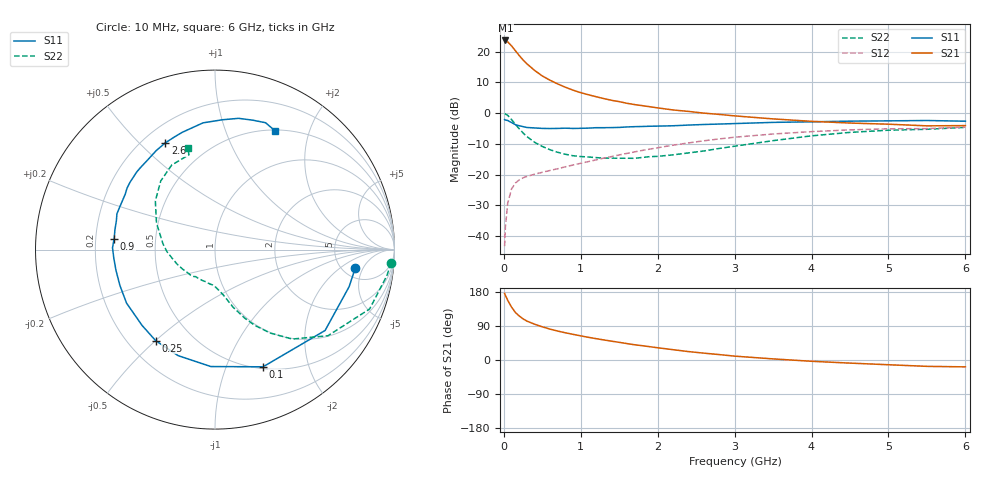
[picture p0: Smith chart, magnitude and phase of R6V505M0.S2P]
! SIEMENS Small Signal Semiconductors
! BFR193
! Si NPN RF Bipolar Junction Transistor in SOT23
! VCE = 0.5 V  IC = 5 mA
! Common Emitter S-Parameters:  May  1996
# GHz  S  MA  R  50
!  f  S11  S21  S12  S22
! GHz  MAG  ANG  MAG  ANG  MAG  ANG  MAG  ANG
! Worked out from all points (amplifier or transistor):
!   36 points, 10 MHz to 6 GHz, reference 50 ohm
!   highest |S21| = 23.6 dB at 20 MHz (marker M1)
!   |S21| within 3 dB of that: start of sweep to 139.3 MHz
!   unconditionally stable (mu >= 1): 849.4 MHz to 2.434 GHz; 5.47 GHz to end of sweep
!   at 250 MHz: K = 0.44, MSG = 19.2 dB, |S12| = -21.0 dB
!   at 1.4 GHz: K = 1.10, MAG = 7.3 dB, |S12| = -14.1 dB
!   at 6 GHz: K = 1.01, MAG = -0.2 dB, |S12| = -4.5 dB
!   S11 on the Smith chart (normalised r, x): 10 MHz: 6.44, -3.54; 100 MHz: 0.52, -1.36; 250 MHz: 0.31, -0.50; 900 MHz: 0.28, +0.05; 2.6 GHz: 0.29, +0.60; 6 GHz: 0.51, +1.50
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0.01  0.7877 -7.6  15.21 175.7  0.0069 85.6  0.9842 -4.3
0.02  0.7755 -15.4  15.22 170.6  0.014 81.1  0.9682 -8.7
0.05  0.7611 -36.3  14.45 157.7  0.0342 71.8  0.9228 -21.0
0.1  0.7058 -67.7  12.43 139.6  0.0585 59.0  0.7916 -37.3
0.15  0.652 -92.0  10.37 125.5  0.0734 50.2  0.6584 -49.2
0.2  0.6254 -109.2  8.661 116.1  0.0824 45.0  0.5575 -56.5
0.25  0.6055 -123.1  7.337 108.5  0.0891 42.2  0.478 -62.2
0.3  0.5861 -133.9  6.351 102.7  0.0938 40.8  0.417 -66.5
0.4  0.576 -148.8  4.962 94.4  0.102 40.1  0.3369 -72.5
0.5  0.5663 -159.3  4.031 87.5  0.1095 40.7  0.288 -76.3
0.6  0.5637 -168.3  3.438 81.5  0.1173 41.9  0.2549 -79.9
0.7  0.5659 -175.4  2.992 76.4  0.1252 43.5  0.2317 -83.9
0.9  0.5652 173.8  2.367 67.7  0.1438 46.1  0.2033 -90.7
1.1  0.5723 163.8  1.994 59.8  0.1636 47.8  0.1941 -97.9
1.3  0.5815 155.6  1.727 52.9  0.1864 48.7  0.186 -106.1
1.6  0.598 145.0  1.449 43.3  0.2222 48.9  0.1855 -120.5
2.2  0.6249 126.8  1.129 27.2  0.3022 44.9  0.2106 -148.9
2.6  0.6557 115.0  1.003 18.1  0.356 40.2  0.2432 -168.5
3.5  0.7093 95.4  0.808 2.9  0.4593 26.2  0.3579 155.6
4.5  0.7431 79.8  0.692 -8.2  0.5361 11.1  0.4877 128.3
5.5  0.7609 68.3  0.623 -16.8  0.562 -3.2  0.5478 105.4
6  0.7413 63.1  0.629 -18.1  0.5938 -7.4  0.5883 104.8
